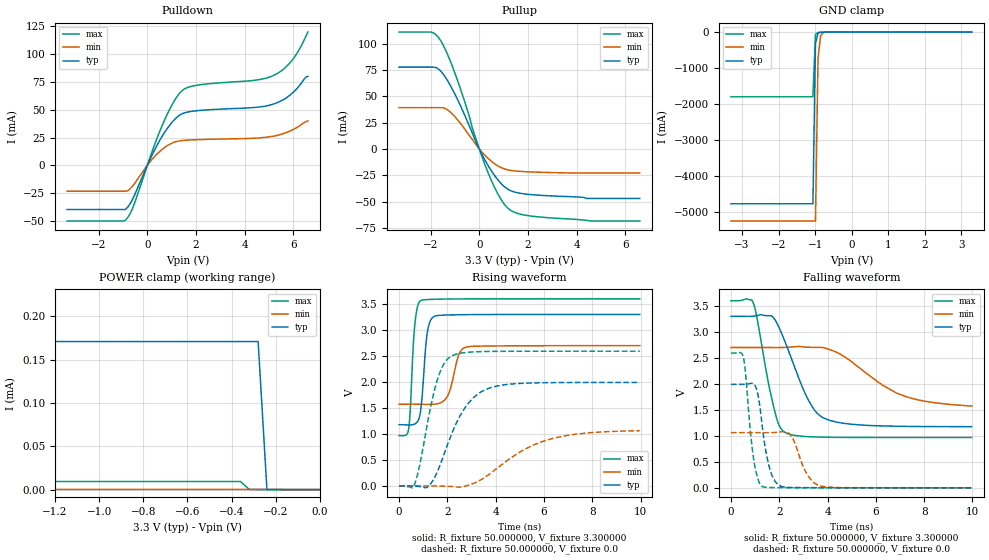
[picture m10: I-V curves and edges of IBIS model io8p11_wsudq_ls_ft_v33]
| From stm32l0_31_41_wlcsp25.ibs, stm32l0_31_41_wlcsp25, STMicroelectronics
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|   Model io8p11_wsudq_ls_ft_v33
[Model]  io8p11_wsudq_ls_ft_v33
Model_type I/O
Polarity   Non-Inverting
Enable   Active-Low
Vinl =   0.990000V
Vinh =   2.310000V
Vmeas =  1.650000V
Cref =   50.000000pF
Rref =   100.000000M
Vref =   0.0V
C_comp   2.653200pF   2.620200pF   2.695100pF
[Temperature Range]   25.000000   0.125000k   -40.000000
[Pullup Reference]   3.300000V   2.700000V   3.600000V
[Pulldown Reference]   0.0V   0.0V   0.0V
[POWER Clamp Reference]   3.300000V   2.700000V   3.600000V
[GND Clamp Reference]   0.0V   0.0V   0.0V
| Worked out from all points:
|   slope of the pulldown table from 0 to 0.495 V, typ, clamps not added: 22.6 ohm
|   slope of the pullup table from 0 to 0.495 V, typ, clamps not added: 23.9 ohm
|   GND clamp passes 1 mA (typ) near -0.64 V on its own axis
|   POWER clamp passes 1 mA (typ) near -2.99 V on its own axis
|   rising waveform, R_fixture 50.000000, V_fixture 3.300000: 20-80 % time 216ps typ, 361ps min, 180ps max; typ from 1.18 V to 3.3 V
|   rising waveform, R_fixture 50.000000, V_fixture 0.0: 20-80 % time 1.18ns typ, 2.22ns min, 704ps max; typ from 0 V to 1.99 V
|   falling waveform, R_fixture 50.000000, V_fixture 3.300000: 20-80 % time 1.13ns typ, 2.15ns min, 648ps max; typ from 3.3 V to 1.18 V
|   falling waveform, R_fixture 50.000000, V_fixture 0.0: 20-80 % time 401ps typ, 571ps min, 321ps max; typ from 1.99 V to 0 V
[Pulldown]
|Voltage   I(typ)   I(min)   I(max)
-3.3V     -39.83mA   -23.37mA   -50.2mA
-900mV    -39.83mA   -23.37mA   -49.53mA
-600mV    -30.28mA   -18.59mA   -38.45mA
500mV     22.11mA    12.28mA    30.1mA
1V        38.33mA    19.81mA    53.88mA
1.4V      46.1mA     22.18mA    66.72mA
2V        49.07mA    23.01mA    71.93mA
4.4V      52.05mA    24.38mA    76.53mA
5.2V      55.25mA    26.3mA     81.02mA
5.9V      63.83mA    31.17mA    93.18mA
6.2V      70.39mA    34.76mA    102.6mA
6.6V      80mA       40mA       120mA
[Pullup]
|Voltage   I(typ)   I(min)   I(max)
-3.3V     77.63mA    39.16mA    110.9mA
-2V       77.63mA    39.16mA    110.9mA
-1.6V     74.23mA    39.16mA    103.2mA
-1.3V     64.66mA    36.99mA    89.44mA
-900mV    47.13mA    27.82mA    65.37mA
-200mV    9.95mA     6.205mA    13.84mA
300mV     -13.29mA   -7.65mA    -18.99mA
800mV     -30.32mA   -16.54mA   -44.19mA
1.2V      -38.62mA   -20mA      -56.79mA
1.6V      -41.75mA   -21.17mA   -61.39mA
2.5V      -43.99mA   -22.16mA   -64.64mA
6.6V      -47mA      -22.8mA    -68.42mA
[GND_clamp]
|Voltage   I(typ)   I(min)   I(max)
-3.3V     -4.766A    -5.244A    -1.797A
-1.06V    -4.766A    -5.244A    -1.797A
-990mV    -326.7mA   -5.244A    -68.05mA
-920mV    -29.09mA   -722.2mA   -11.16mA
-850mV    -6.797mA   -104.4mA   -6.682mA
-780mV    -3.554mA   -17.44mA   -4.265mA
-500mV    -58.08uA   -169.3uA   -34.1uA
3.28V     0A         0A         0A
[POWER_clamp]
|Voltage   I(typ)   I(min)   I(max)
-3.28V    3.05A      15.65uA    3.723A
-3.2V     3.05A      1.687uA    3.723A
-2.96V    269.4uA    209.1nA    3.723A
-2.92V    170.9uA    209.1nA    508.5mA
-2.8V     170.9uA    209.1nA    1.296mA
-2.76V    170.9uA    209.1nA    177.1uA
-2.72V    170.9uA    209.1nA    24.25uA
-2.68V    170.9uA    209.1nA    9.362uA
-360mV    170.9uA    209.1nA    9.362uA
-280mV    170.9uA    209.1nA    0A
-240mV    0A         209.1nA    0A
0V        0A         0A         0A
[Ramp]
| variable   typ   min   max
dV/dt_r  1.19472/1.17728n   0.62652/2.18456n   1.55562/0.70290n
dV/dt_f  1.27320/1.12771n   0.63300/2.05394n   1.57853/0.64669n
R_load = 50.000000
[Rising Waveform]
R_fixture= 50.000000
V_fixture= 3.300000
V_fixture_min= 2.700000
V_fixture_max= 3.600000
|time   V(typ)   V(min)   V(max)
0s        1.177V     1.573V     968.4mV
400.4ps   1.173V     1.574V     1.098V
640.6ps   1.19V      1.574V     3.038V
900.9ps   1.467V     1.572V     3.567V
1.161ns   2.92V      1.569V     3.587V
1.461ns   3.263V     1.571V     3.592V
2.022ns   3.289V     1.738V     3.597V
2.462ns   3.294V     2.509V     3.599V
2.803ns   3.296V     2.673V     3.599V
9.97ns    3.3V       2.7V       3.6V
[Rising Waveform]
R_fixture= 50.000000
V_fixture= 0.0
V_fixture_min= 0.0
V_fixture_max= 0.0
|time   V(typ)   V(min)   V(max)
0s        233.5uV    13.27uV    8.59uV
640.6ps   -5.597mV   200.4uV    30.63mV
1.141ns   -32.41mV   47.67uV    1.115V
1.542ns   226.3mV    -1.963mV   1.968V
1.842ns   580.6mV    -5.498mV   2.336V
2.162ns   981mV      -11.15mV   2.496V
2.843ns   1.575V     9.268mV    2.571V
3.864ns   1.9V       269.2mV    2.589V
6.386ns   1.988V     915.5mV    2.592V
9.97ns    1.992V     1.062V     2.593V
[Falling Waveform]
R_fixture= 50.000000
V_fixture= 3.300000
V_fixture_min= 2.700000
V_fixture_max= 3.600000
|time   V(typ)   V(min)   V(max)
0s        3.3V       2.7V       3.6V
920.9ps   3.304V     2.7V       3.56V
1.061ns   3.313V     2.7V       3.312V
1.802ns   3.246V     2.7V       1.495V
2.002ns   3.074V     2.699V     1.198V
2.242ns   2.809V     2.702V     1.066V
3.163ns   1.73V      2.706V     985.6mV
3.884ns   1.335V     2.691V     974.7mV
6.847ns   1.185V     1.826V     968.7mV
9.97ns    1.177V     1.573V     968.4mV
[Falling Waveform]
R_fixture= 50.000000
V_fixture= 0.0
V_fixture_min= 0.0
V_fixture_max= 0.0
|time   V(typ)   V(min)   V(max)
0s        1.992V     1.062V     2.593V
520.5ps   1.991V     1.062V     2.501V
940.9ps   2V         1.062V     547.7mV
1.121ns   1.786V     1.062V     166mV
1.301ns   1.165V     1.062V     26.22mV
1.662ns   286.1mV    1.062V     6.437mV
2.142ns   21.2mV     1.081V     4.042mV
2.482ns   7.142mV    1.005V     2.918mV
3.644ns   2.764mV    45.24mV    852.2uV
9.97ns    233.5uV    13.27uV    8.59uV
